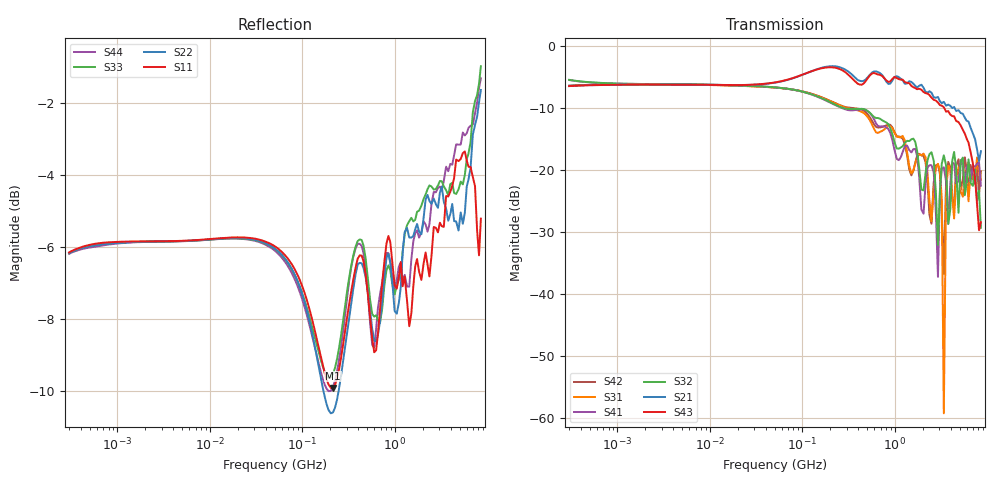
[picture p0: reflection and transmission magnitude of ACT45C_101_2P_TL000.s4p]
! S-Parameter Data Generated by TDK Corporation
! Copyright(C) 2025 TDK Corporation.
! All Rights Reserved.
! TDK P/N: ACT45C-101-2P-TL000 (Signal Line Common Mode Choke/Filter)
! Property: |Zc|=5800ohm at 10MHz
! Size(LxWxT): 4.5x3.2x2.8mm
! Model Type: s2p (Touchstone File Format Version 1.0)
! Frequency: DC=Yes Start=0.3MHz Stop=8500MHz 202points Log-sweep
! Model Generated on July 30, 2025
! Terms and conditions regarding TDK Simulation Models:
! 1)This simulation model is being provided solely for informational
!  purposes. Please refer to the specifications of the products in
!  terms of detailed characteristics of such products.
! 2)In no event shall TDK Corporation of any of its subsidiaries be
!  liable for any loss or damage arising, directly or indirectly,
!  from any information contained in this simulation model, including,
!  but not limited to loss or damages arising from any inaccuracies,
!  omissions or errors in connection with such information.
! 3)Any and all copyrights on this simulation model are owned by
!  TDK Corporation.  Duplication or redistribution of this simulation
!  model without prior written permission from TDK Corporation
!  is prohibited.
! 4)This simulation model is subject to any modification or change
!  without any prior notice.
! 5)Neither TDK Corporation nor any of its subsidiaries shall make any
!  warranty, express or implied, including but not limited to the
!  correctness, implied warranties of merchantability and fitness for
!  a particular purpose with respect to this simulation models.
! 6)The use of this simulation model shall be deemed to have consented
!  to the terms and conditions hereof.
! Port Assignments:
!  1 ---@@@--- 4
!  2 ---@@@--- 3
! Applicable Conditions:
!  Temperature = 25 degC
!  DC Bias Current = 0 A
!  Small Signal Operation
# Hz S MA R 50
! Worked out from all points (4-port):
!   201 points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, 300 kHz to 8.5 GHz, reference 50 ohm
!   strongest paths, dB at 300 kHz, 3.892 MHz, 50.5 MHz, 655.2 MHz, 8.5 GHz:
!     S43: -6.5, -6.2, -5.9, -4.6, -28.4
!     S21: -6.4, -6.2, -5.9, -4.2, -17.0
!     S32: -5.5, -6.2, -6.7, -11.6, -29.3
!     S41: -5.5, -6.2, -6.7, -12.9, -22.5
!     S31: -6.4, -6.2, -6.7, -14.0, -21.6
!     S42: -6.5, -6.2, -6.7, -13.1, -20.2
!   lowest |S11| = -9.9 dB at 213.8 MHz (marker M1), VSWR 1.94, Z = 96.7 - j2.71 ohm
!   |S11| at or under -10 dB: nowhere
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300000  0.492 13.0  0.479 13.7  0.4783 -166.6  0.5366 -12.2
        0.4793 13.8  0.4906 13.0  0.5355 -12.9  0.4806 -165.8
        0.4782 -165.9  0.5337 -12.4  0.4913 13.2  0.4798 14.8
        0.5321 -12.4  0.4749 -165.9  0.4757 14.2  0.4898 14.3
2.138282e8  0.3189 -2.3  0.6881 -5.6  0.3495 69.3  0.3392 -112.8
            0.688 -5.8  0.2949 -1.2  0.3416 -112.4  0.3508 66.0
            0.3513 69.1  0.3435 -112.3  0.3334 3.4  0.672 -8.1
            0.3411 -112.9  0.3528 66.2  0.6723 -8.0  0.3198 3.9
2.91934e9  0.5246 -52.3  0.3875 -61.4  0.112 37.0  0.01405 107.1
           0.3877 -61.8  0.5674 -48.5  0.02241 -146.1  0.1116 38.4
           0.1121 35.2  0.02486 -143.2  0.6094 -46.6  0.3453 -69.4
           0.01374 105.9  0.1107 36.8  0.3502 -68.3  0.6048 -50.1
3.209598e9  0.5351 -56.8  0.346 -62.9  0.05764 -33.7  0.1022 48.6
            0.3461 -63.2  0.6072 -55.4  0.1124 77.8  0.04733 -29.6
            0.05872 -34.9  0.1124 78.1  0.6177 -51.7  0.3285 -72.6
            0.102 47.1  0.04703 -31.1  0.3306 -72.7  0.6001 -54.9
3.378408e9  0.5338 -55.5  0.3567 -66.8  0.001456 123.6  0.1051 19.5
            0.3545 -65.3  0.5785 -58.1  0.1305 39.0  0.01449 94.2
            0.001089 161.4  0.1314 38.1  0.6076 -54.1  0.3206 -76.7
            0.105 19.2  0.01454 92.7  0.3212 -77.0  0.6186 -53.9
3.773187e9  0.5884 -64.3  0.3378 -70.5  0.1077 32.7  0.03617 15.3
            0.3369 -70.2  0.5445 -64.4  0.03573 -29.7  0.1142 30.2
            0.1079 33.4  0.03674 -27.9  0.5908 -59.2  0.3019 -81.2
            0.03674 14.9  0.1163 29.8  0.2986 -81.4  0.6378 -61.5
8.5e9  0.5481 -166.0  0.1416 -160.8  0.07849 -117.5  0.077 -114.6
       0.1417 -161.0  0.8271 -93.0  0.03301 -96.3  0.1003 -68.4
       0.08343 -106.8  0.03417 -85.4  0.8925 -95.7  0.03557 -102.6
       0.07483 -105.1  0.09769 -58.8  0.03791 -113.7  0.8586 -132.8
